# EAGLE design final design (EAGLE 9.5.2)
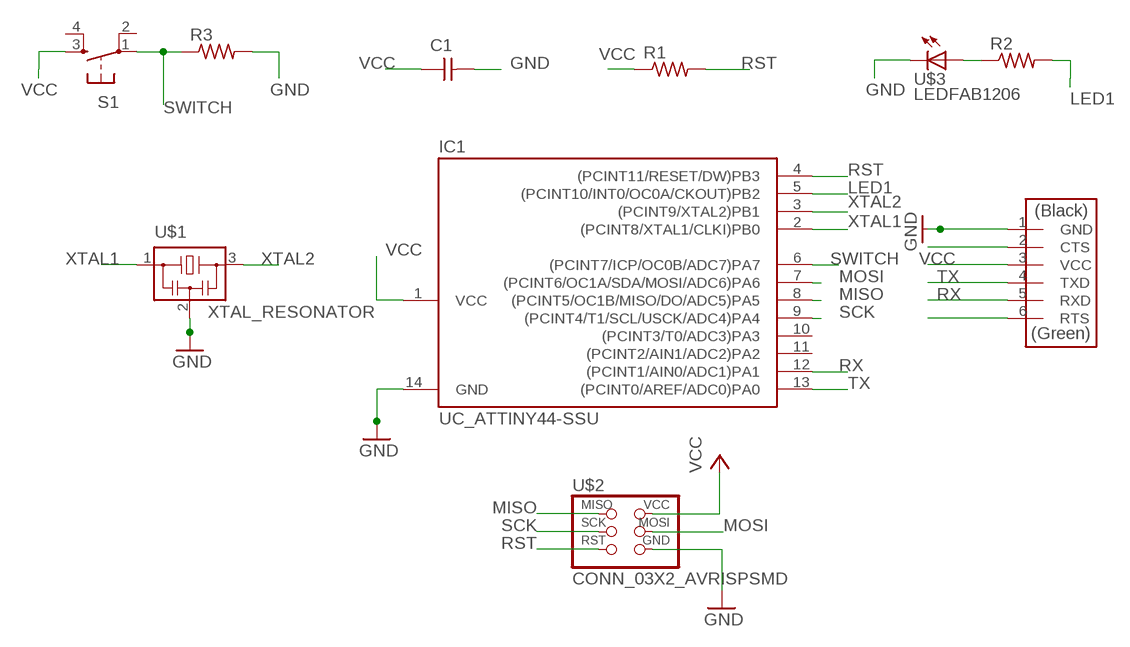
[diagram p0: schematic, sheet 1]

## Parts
C1  CAP_UNPOLARIZEDFAB  [C1206FAB]
IC1  UC_ATTINY44-SSU  [SOIC14]
R1  R1206FAB  [R1206FAB]
R2  R1206FAB  [R1206FAB]
R3  R1206FAB  [R1206FAB]
S1  SW_SWITCH_TACTILE_6MM6MM_SWITCH  [6MM_SWITCH]
U$1  XTAL_RESONATOR  [EFOBM]
U$2  CONN_03X2_AVRISPSMD  [2X03SMD]
U$3  LEDFAB1206  [LED1206FAB]
U$4  CONN_06_FTDI-SMD-HEADER  [1X06SMD]

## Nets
GND: C1.2 IC1.14(GND) R3.2 U$1.2 U$2.6(GND) U$3.2(C) U$4.1(GND)
LED1: IC1.5((PCINT10/INT0/OC0A/CKOUT)PB2) R2.2
MISO: IC1.8((PCINT5/OC1B/MISO/DO/ADC5)PA5) U$2.1(MISO)
MOSI: IC1.7((PCINT6/OC1A/SDA/MOSI/ADC6)PA6) U$2.4(MOSI)
N$2: R2.1 U$3.1(A)
N$6: U$4.2(CTS)
N$10: U$4.6(RTS)
RST: IC1.4((PCINT11/RESET/DW)PB3) R1.2 U$2.5(RST)
RX: IC1.12((PCINT1/AIN0/ADC1)PA1) U$4.5(RXD)
SCK: IC1.9((PCINT4/T1/SCL/USCK/ADC4)PA4) U$2.3(SCK)
SWITCH: IC1.6((PCINT7/ICP/OC0B/ADC7)PA7) R3.1 S1.1(P)
TX: IC1.13((PCINT0/AREF/ADC0)PA0) U$4.4(TXD)
VCC: C1.1 IC1.1(VCC) R1.1 S1.3(S) U$2.2(VCC) U$4.3(VCC)
XTAL1: IC1.2((PCINT8/XTAL1/CLKI)PB0) U$1.1
XTAL2: IC1.3((PCINT9/XTAL2)PB1) U$1.3
Unconnected: IC1.10((PCINT3/T0/ADC3)PA3) IC1.11((PCINT2/AIN1/ADC2)PA2) S1.2(P1) S1.4(S1)

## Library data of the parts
C1 = fab:CAP_UNPOLARIZED
IC1 = fab:UC_ATTINY44
R1-R3 = fab:R: Resistor (US Symbol)
S1 = fab:SW_SWITCH_TACTILE_6MM: OMRON SWITCH
U$1 = fab:XTAL_RESONATOR
U$2 = fab:CONN_03X2_AVRISP
U$3 = fab:LED: LED
U$4 = fab:CONN_06_FTDI-SMD-HEADER

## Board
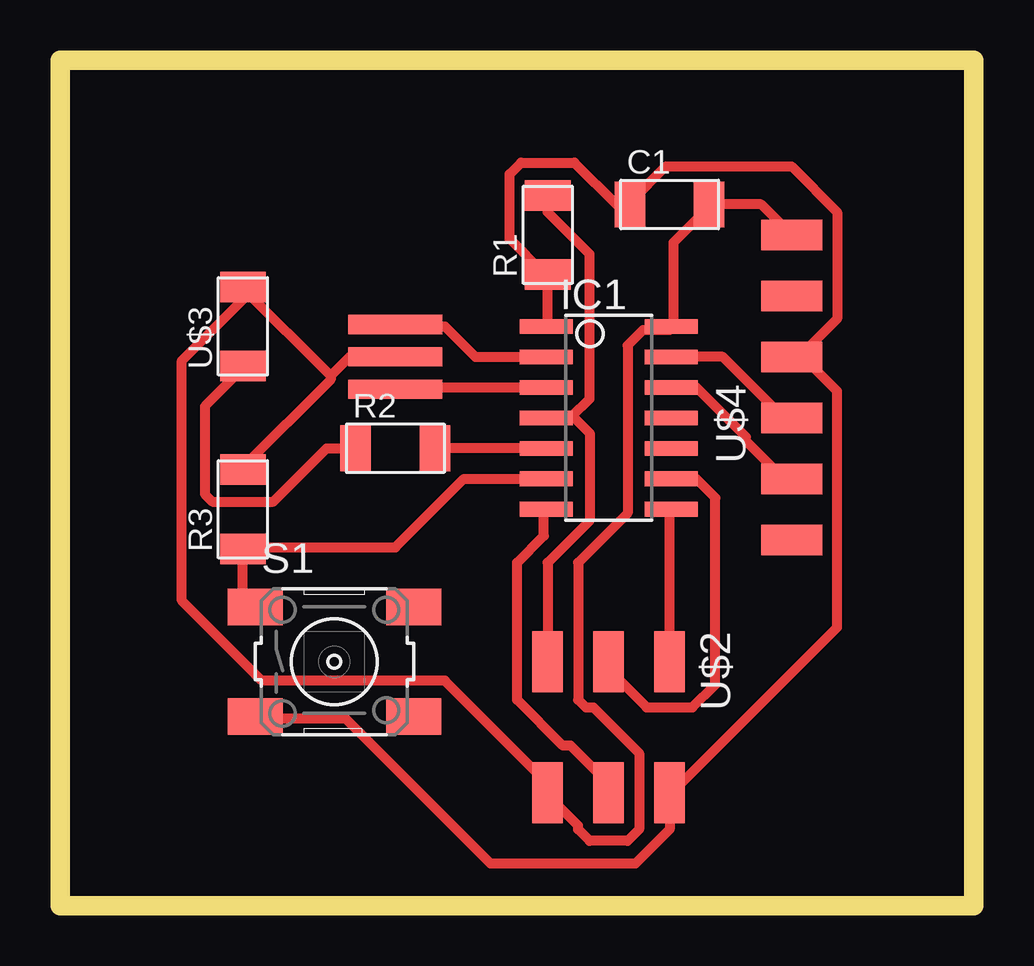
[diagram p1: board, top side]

Size 38.08 x 35.23 mm. Coordinates in mm from the lower left corner, seen from the top.
Outline: 0,0 38.08,0 38.08,35.23 0,35.23 0,0
Copper layers (1*16): Top 0.035mm / dielectric 1.5mm / Bottom 0.035mm
Design rules "default *": minimum track width 16mil, minimum drill 0.35mm, track to track 16mil, track to pad 16mil, pad to pad 16mil, via to via 16mil, smd to smd 16mil, copper to edge 40mil, drill to drill 16mil, minimum pad ring 10mil, minimum via ring 8mil, stop-mask expansion 4mil, vias tented up to drill 0mil, thermal gap 10mil

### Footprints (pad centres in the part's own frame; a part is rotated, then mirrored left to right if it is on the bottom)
C1206FAB = smd 1.27 x 1.905: 1 -1.651,0; 2 1.651,0
SOIC14 = smd 0.61 x 2.21: 1 -3.81,-2.603; 2 -2.54,-2.603; 3 -1.27,-2.603; 4 0,-2.603; 5 1.27,-2.603; 6 2.54,-2.603; 7 3.81,-2.603; 8 3.81,2.603; 9 2.54,2.603; 10 1.27,2.603; 11 0,2.603; 12 -1.27,2.603; 13 -2.54,2.603; 14 -3.81,2.603
R1206FAB = smd 1.27 x 1.905: 1 -1.651,0; 2 1.651,0
6MM_SWITCH = smd 2.286 x 1.524: 1 -3.302,2.286; 2 3.302,2.286; 3 -3.302,-2.286; 4 3.302,-2.286
EFOBM = smd 0.8 x 3.9: 1 -1.35,0; 2 0,0; 3 1.35,0
2X03SMD = smd 2.54 x 1.27: 1 -2.54,2.54; 2 2.92,2.54; 3 -2.54,0; 4 2.92,0; 5 -2.54,-2.54; 6 2.92,-2.54
LED1206FAB = smd 1.27 x 1.905: 1 -1.651,0; 2 1.651,0
1X06SMD = smd 2.54 x 1.27: 1 0,6.35; 2 0,3.81; 3 0,1.27; 4 0,-1.27; 5 0,-3.81; 6 0,-6.35

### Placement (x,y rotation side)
C1  25.4,29.21 0 top
IC1  22.86,20.32 270 top
R1  20.32,27.94 90 top
R2  13.97,19.05 0 top
R3  7.62,16.51 90 top
S1  11.43,10.16 0 top
U$1  13.97,22.86 270 top
U$2  22.86,7.62 270 top
U$3  7.62,24.13 90 top
U$4  30.48,21.59 0 top

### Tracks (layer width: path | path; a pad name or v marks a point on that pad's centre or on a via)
GND
  Top 0.406: 11.27,22.07 12.06,22.86 U$1.2 | R3.2 7.62,18.26 11.27,21.91 11.27,22.07 | 11.27,22.07 7.62,25.72 U$3.2 7.78,25.4 5.08,22.7 5.08,12.7 8.41,9.37 16.03,9.37 20.16,5.24 20.16,4.76 U$2.6 20.32,4.6 21.59,3.33 21.59,3.18 22.07,2.7 23.65,2.7 24.13,3.18 24.13,6.35 22.23,8.26 21.91,8.26 21.59,8.57 21.59,14.29 23.65,16.35 23.65,23.34 24.29,23.97 25.4,23.97 IC1.14 25.56,24.13 25.56,27.62 26.99,29.05 C1.2 29.21,29.21 U$4.1
LED1
  Top 0.406: IC1.5 R2.2
MISO
  Top 0.406: U$2.1 25.4,16.51 IC1.8
MOSI
  Top 0.406: U$2.4 22.86,5.08 21.27,6.67 20.95,6.67 19.05,8.57 19.05,14.29 20.16,15.4 20.16,16.51 IC1.7
N$2
  Top 0.406: R2.1 11.11,19.05 8.89,16.83 6.35,16.83 6.03,17.14 6.03,20.8 7.62,22.38 U$3.1
RST
  Top 0.406: R1.2 20.32,28.89 22.07,27.15 22.07,21.11 21.35,20.4 | 21.35,20.4 21.27,20.32 IC1.4 | U$2.5 20.32,14.29 22.07,16.03 22.07,19.68 21.35,20.4
RX
  Top 0.406: IC1.12 26.51,21.59 28.58,19.53 28.58,19.37 30.16,17.78 U$4.5
SCK
  Top 0.406: IC1.9 26.51,17.78 27.3,16.99 27.3,9.21 26.35,8.26 24.45,8.26 22.86,9.84 U$2.3
SWITCH
  Top 0.406: S1.1 8.1,12.54 7.62,13.02 R3.1 7.78,14.92 13.97,14.92 16.83,17.78 IC1.6
TX
  Top 0.406: IC1.13 27.62,22.86 30.16,20.32 U$4.4
VCC
  Top 0.406: IC1.1 20.32,24.13 R1.1 20.16,26.35 18.73,27.78 18.73,30.48 19.21,30.96 21.43,30.96 23.18,29.21 C1.1 23.81,29.37 25.24,30.8 30.48,30.8 32.39,28.89 32.39,24.45 30.8,22.86 U$4.3 30.96,22.86 32.39,21.43 32.39,11.59 25.56,4.76 U$2.2 25.4,3.18 23.97,1.75 17.94,1.75 11.91,7.78 8.22,7.78 S1.3
XTAL1
  Top 0.406: IC1.2 17.3,22.86 16.03,24.13 13.97,24.13 U$1.1
XTAL2
  Top 0.406: IC1.3 13.97,21.59 U$1.3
